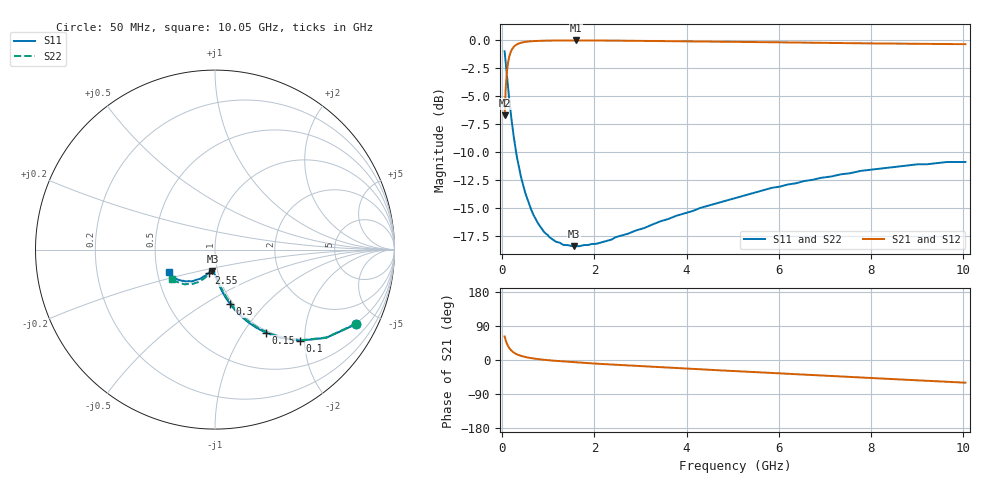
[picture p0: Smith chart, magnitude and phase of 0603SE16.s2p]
! AVX Thin Film Operation		Date: August 2001
! Description: Accu-P® Series, Thin Film, SMD, RF Capacitor
! Part Number: 06033J160FBT
! 50 MHz  -  10.05 GHz
! Serial Measurements
# mhz S db R 50
!	S11		S21		S12		S22
!	dB	Phase	dB	Phase	dB	Phase	dB	Phase
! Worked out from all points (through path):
!   401 points, 50 MHz to 10.05 GHz, reference 50 ohm
!   highest |S21| = -0.07 dB at 1.6 GHz (marker M1); lowest = -6.8 dB at 50 MHz (marker M2)
!   group delay of S21, straight-line fit = 19.6 ps
!   lowest |S11| = -18.4 dB at 1.55 GHz (marker M3), VSWR 1.27, Z = 47.2 - j11.4 ohm
!   |S11| at or under -10 dB: 298.4 MHz to end of sweep
!   |S22| runs from -18.4 to -1.0 dB; largest |S21 - S12| = 0.00011
!   S11 on the Smith chart (normalised r, x): 50 MHz: 0.96, -3.80; 100 MHz: 0.97, -1.90; 150 MHz: 0.97, -1.27; 300 MHz: 0.97, -0.65; 2.55 GHz: 0.90, -0.24; 10.05 GHz: 0.58, -0.16
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50  -1.03 -27.9  -6.75 62.2  -6.75 62.2  -1.03 -27.7
100  -3.16 -46.9  -2.88 43.2  -2.88 43.2  -3.16 -46.6
125  -4.25 -53.4  -2.05 36.8  -2.05 36.8  -4.25 -53.0
150  -5.30 -58.5  -1.53 31.7  -1.53 31.7  -5.30 -58.0
175  -6.24 -62.5  -1.18 27.8  -1.18 27.8  -6.24 -62.0
225  -7.94 -68.5  -0.77 21.8  -0.77 21.8  -7.94 -67.8
300  -10.04 -74.4  -0.46 15.9  -0.46 15.9  -10.04 -73.6
400  -12.13 -79.4  -0.28 11.1  -0.28 11.1  -12.13 -78.2
500  -13.68 -82.7  -0.20 7.8  -0.20 7.8  -13.68 -81.4
650  -15.36 -86.2  -0.13 4.5  -0.13 4.5  -15.36 -84.5
775  -16.36 -88.4  -0.11 2.4  -0.11 2.4  -16.36 -86.4
925  -17.22 -90.5  -0.09 0.3  -0.09 0.3  -17.22 -88.3
1125  -17.89 -92.8  -0.08 -1.9  -0.08 -1.9  -17.89 -90.4
1550  -18.40 -96.9  -0.07 -5.8  -0.07 -5.8  -18.40 -94.0
1600  -18.40 -97.3  -0.07 -6.2  -0.07 -6.2  -18.40 -94.4
1725  -18.35 -98.4  -0.07 -7.2  -0.07 -7.2  -18.35 -95.4
2550  -17.50 -105.0  -0.09 -13.2  -0.09 -13.2  -17.50 -101.0
3400  -16.23 -109.9  -0.11 -18.9  -0.11 -18.9  -16.23 -106.9
5050  -14.12 -121.4  -0.19 -29.4  -0.19 -29.4  -14.02 -116.4
6725  -12.49 -132.0  -0.27 -39.6  -0.27 -39.6  -12.40 -126.0
8400  -11.39 -143.1  -0.35 -49.9  -0.35 -49.9  -11.39 -136.1
10050  -10.90 -153.6  -0.40 -59.9  -0.40 -59.9  -10.82 -145.8
